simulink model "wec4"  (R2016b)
settings: Solver=ode4  StartTime=0  StopTime=1000  FixedStep=0.005  MaxStep=0.005  RelTol=1e-3  EnableMultiTasking=on
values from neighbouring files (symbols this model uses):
  arAdaptiveLawData = 1/2*zModelSimple.zModelPto.arFreq.*     zModelSimple.zModelPto.arMagnitude./     cos(zModelSimple.zModelPto.arPhase*pi/180+pi/2)    [IMPACT_Control.m]
  arAdaptiveLawDataX = 1/2*zModelSimpleX.zModelPto.arFreq.*         zModelSimpleX.zModelPto.arMagnitude./         cos(zModelSimpleX.zModelPto.arPhase*pi/180+pi/2)    [IMPACT_Control.m]
  arControllerRampGain = [0,0,1,1]    [IMPACT_Control.m]
  arControllerRampTime = [0 rStartRampTime rStartRampTime+rRampTimeLength 8000]    [IMPACT_Control.m]
  arEkfInitialisation = zeros(1,11)    [IMPACT_Control.m]
  arEkfInitialisationX = zeros(1,11)    [IMPACT_Control.m]
  arFrequency = zModelSimple.zModelPto.arFreq    [IMPACT_Control.m]
  arFrequencyRange = zModelSimple.zModelPto.arFreq    [IMPACT_Control.m]
  arFrequencyX = zModelSimpleX.zModelPto.arFreq    [IMPACT_Control.m]
  arImpedance = 1./zModelSimple.zModelPto.arMagnitude./zModelSimple.zModelPto.arFreq    [IMPACT_Control.m]
  arImpedanceX = 1./zModelSimpleX.zModelPto.arMagnitude./zModelSimpleX.zModelPto.arFreq    [IMPACT_Control.m]
  CentralPTOPreload = -1.6113e+07    (= -16113000)    [wecSimInputFile.m]
  F1 = [4.243 2.375 -12.243]    [wecSimInputFile.m]
  F2 = [4.243 -2.375 -12.243]    [wecSimInputFile.m]
  F3 = [-4.243 -2.375 -12.243]    [wecSimInputFile.m]
  F4 = [-4.243 2.375 -12.243]    [wecSimInputFile.m]
  FC = [0 0 -14]    [wecSimInputFile.m]
  iAdaptiveDamping = 0    [wec4IMPACT_Project.m]    (also in IMPACT_Control.m = handles.iAdaptiveDamping; wec1_IMPACT_Project.m; wec2_IMPACT_Project.m; wec3_IMPACT_Project.m)
  iControlType = 2    [wec4IMPACT_Project.m]    (also in IMPACT_Control.m = handles.iControlType; wec1_IMPACT_Project.m = 1; wec2_IMPACT_Project.m = 1; wec3_IMPACT_Project.m = 1)
  iPtoPositionConstraint = 1    [wec4IMPACT_Project.m]    (also in IMPACT_Control.m = handles.iPtoPositionConstraint; wec1_IMPACT_Project.m = 0; wec2_IMPACT_Project.m; wec3_IMPACT_Project.m)
  iSensorNoise = 0    [IMPACT_Control.m]
  m = m+1    (= 2)    [checkParamFile.m]
  PTOrotation = atan((T1(2)-F1(2))/(T1(1)-F1(1)))    [wecSimInputFile.m]
  rCogFloater = -8    [wec4_IMPACT_Model.m]    (also in paramInitial.m = get( handles.edit_rCogFloater, 'String' ); wec1_IMPACT_Model.m = -18; wec2_IMPACT_Model.m = -8.5; wec3_IMPACT_Model.m = -0.7)
  rCogSpar = -36.6    [wec4_IMPACT_Model.m]    (also in paramInitial.m = get( handles.edit_rCogSpar, 'String' ); wec3_IMPACT_Model.m = -21.3; wec3_IMPACT_Model2.m = -21.3)
  rDisplacementLimit = 10.000000    (= 10)    [wec4IMPACT_Project.m]    (also in IMPACT_Control.m = getValue(handles.edit_displacementLimit); wec1_IMPACT_Project.m; wec2_IMPACT_Project.m; wec3_IMPACT_Project.m = 3)
  rDisplacementLimitX = 10.000000    (= 10)    [wec4IMPACT_Project.m]    (also in IMPACT_Control.m = getValue(handles.edit_displacementLimitX); wec1_IMPACT_Project.m = 0; wec2_IMPACT_Project.m; wec3_IMPACT_Project.m = 0)
  rGainForAntiWIndUp = tfControllerDiscrete.rGain    [IMPACT_Control.m]
  rGainForAntiWIndUpX = tfControllerXDiscrete.rGain    [IMPACT_Control.m]
  rMaxForcePto = 300000000.000000    (= 300000000)    [wec4IMPACT_Project.m]    (also in IMPACT_Control.m = getValue(handles.edit_maxForcePto); wec1_IMPACT_Project.m = 1e+15; wec2_IMPACT_Project.m = 1e+15; wec3_IMPACT_Project.m = 1000000000)
  rMinForcePto = -300000000.000000    (= -300000000)    [wec4IMPACT_Project.m]    (also in IMPACT_Control.m = getValue(handles.edit_minForcePto); wec1_IMPACT_Project.m = -1e+15; wec2_IMPACT_Project.m = -1e+15; wec3_IMPACT_Project.m = -1000000000)
  rMooringX = 20000    [wec4_IMPACT_Model.m]    (also in paramInitial.m = get( handles.edit_rMooringX, 'String' ); wec3_IMPACT_Model.m = 10000; wec3_IMPACT_Model2.m = 10000)
  rMooringZ = 10000    [wec4_IMPACT_Model.m]    (also in paramInitial.m = get( handles.edit_rMooringZ, 'String' ); wec3_IMPACT_Model.m = 0; wec3_IMPACT_Model2.m = 0)
  rOutputSampleTime = 0.010000    (= 0.01)    [wec4IMPACT_Project.m]    (also in IMPACT_Control.m = getValue(handles.edit_outputSampleTime); wec1_IMPACT_Project.m; wec2_IMPACT_Project.m; wec3_IMPACT_Project.m)
  rPassiveDampingGain = -604830.000000    (= -604830)    [wec4IMPACT_Project.m]    (also in IMPACT_Control.m = getValue(handles.edit_gainPLD); wec1_IMPACT_Project.m = -214018.1537; wec2_IMPACT_Project.m = -1948070; wec3_IMPACT_Project.m = -519390)
  rPassiveDampingGainX = -278660.000000    (= -278660)    [wec4IMPACT_Project.m]    (also in IMPACT_Control.m = getValue(handles.edit_gainPLDX); wec1_IMPACT_Project.m = 0; wec2_IMPACT_Project.m = 0; wec3_IMPACT_Project.m = 0)
  rTetherPretension = 1.6113e+07    (= 16113000)    [wec4_IMPACT_Model.m]    (also in paramInitial.m = get( handles.edit_rTetherPretension, 'String' ); wec3_IMPACT_Model.m = 0; wec3_IMPACT_Model2.m = 0)
  rTetherSpring = 500000    [wec4_IMPACT_Model.m]    (also in paramInitial.m = get( handles.edit_rTetherSpring, 'String' ); wec3_IMPACT_Model.m = 0; wec3_IMPACT_Model2.m = 0)
  rUpperFrequencyLimit = EKFFloater.upperFreq    [IMPACT_Control.m]
  rXf = 4.243    [wec4AdditionalParams.m]
  rXs = 16.075    [wec4AdditionalParams.m]
  rYf = 2.375    [wec4AdditionalParams.m]
  rYs = 16.075    [wec4AdditionalParams.m]
  rZf = 4.243    [wec4AdditionalParams.m]
  rZs = 2.4350    (= 2.435)    [wec4AdditionalParams.m]
  rZTetherF = 6    [wec4AdditionalParams.m]
  rZTetherS = 2.4350    (= 2.435)    [wec4AdditionalParams.m]
  s = tf('s')    [wec4_IMPACT_Model.m]    (also in IMPACT_Control.m; wec1_IMPACT_Model.m; wec2_IMPACT_Model.m; wec3_IMPACT_Model.m)
  SidePTO1Preload = PreloadPTOCorner    (= 0)    [wecSimInputFile.m]
  SidePTO2Preload = PreloadPTOCorner    (= 0)    [wecSimInputFile.m]
  SidePTO3Preload = PreloadPTOCorner    (= 0)    [wecSimInputFile.m]
  SidePTO4Preload = PreloadPTOCorner    (= 0)    [wecSimInputFile.m]
  simu = simulationClass()    [wecSimInputFile.m]
  T1 = [16.075 16.075 -34.165]    [wecSimInputFile.m]
  T2 = [16.075 -16.075 -34.165]    [wecSimInputFile.m]
  T3 = [-16.075 -16.075 -34.165]    [wecSimInputFile.m]
  T4 = [-16.075 16.075 -34.165]    [wecSimInputFile.m]
  TC = [0 0 -34.165]    [wecSimInputFile.m]
  waves = waveClass('irregular')    [wecSimInputFile.m]
  Z = magPhaseToComplex(zModelTf)    [IMPACT_Control.m]
undefined symbols (not defined in the file or in its folder): arControllerDiscreteDen, arControllerDiscreteNum, arControllerDiscreteXDen, arControllerDiscreteXNum, arExcForceFloaterDen, arExcForceFloaterNum, arExcForceFloaterXDen, arExcForceFloaterXNum, arExcForceSparDen, arExcForceSparNum, arExcForceSparXDen, arExcForceSparXNum, arFexcFloaterDen, arFexcFloaterNum, arFexcFloaterXDen, arFexcFloaterXNum, arFexcSparDen, arFexcSparNum, arFexcSparXDen, arFexcSparXNum, Body, body, constraint, CTTime, deg, Elements, geometry, IRKB, kg, lenJ, mooring, N, pto, rAccelerationGainFloater, rAccelerationGainFloaterX, rAccelerationGainSpar, rAccelerationGainSparX, rad, rBuoyancyGainFloater, rBuoyancyGainFloaterX, rBuoyancyGainSpar, rBuoyancyGainSparX, rDampingGainFloater, rDampingGainFloaterX, rDampingGainSpar, rDampingGainSparX, Rigid, rMaxFocePto, wec4_float, wec4_reactor, WECSim_Lib, X, Y
libraries: nesl_utility x380, sm_lib x170, vrlib x91, simulink x12, WECSim_Lib x4
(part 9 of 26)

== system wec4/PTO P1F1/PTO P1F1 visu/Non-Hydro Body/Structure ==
  Total Force : Inport
  Body Properties : sm_lib/Body Elements/Solid  InertiaType=Custom  Mass=body.mass  MassUnits=kg  CenterOfMass=[0 0 0]  CenterOfMassUnits=m  MomentsOfInertia=body.momOfInertia  MomentsOfInertiaUnits=kg*m^2  ProductsOfInertia=[0 0 0]  ProductsOfInertiaUnits=kg*m^2  DensityBased=on  Density=1000  DensityUnits=kg/(m^3)  DoExposeReferenceFrame=on  SerializedFrames=<Frames/>  GraphicType=FromGeometry  MarkerShape=Sphere  MarkerSize=10  MarkerSizeUnits=m  GraphicVisPropType=SimpleVisualProperties  GraphicDiffuseColor=body.viz.color  GraphicSpecularColor=[0.5 0.5 0.5 1.0]  GraphicAmbientColor=[0.15 0.15 0.15 1.0]  GraphicEmissiveColor=[0.0 0.0 0.0 1.0]  GraphicShininess=75  GraphicOpacity=body.viz.opacity  GeometryShape=FromFile  RectangleSize=[1 1]  RectangleSizeUnits=m  BrickDimensions=[1 1 1]  BrickDimensionUnits=m  CylinderRadius=1  CylinderRadiusUnits=m  CylinderLength=1  CylinderLengthUnits=m  SphereRadius=1  SphereRadiusUnits=m  EllipsoidRadii=[1 1 1]  EllipsoidRadiiUnits=m  ExtrusionCrossSection=[1 1; -1 1; -1 -1; 1 -1]  ExtrusionCrossSectionUnits=m  ExtrusionLength=1  ExtrusionLengthUnits=m  PolygonNumSides=3  PolygonOuterRadius=1  PolygonOuterRadiusUnits=m  ExtGeomFileType=STL  ExtGeomFileName=.\geometry\pto_visu.stl  ExtGeomFileUnits=m  RevolutionCrossSection=[1 1; 1 -1; 2 -1; 2 1]  RevolutionCrossSectionUnits=m  RevolutionExtent=Full  RevolutionAngle=180  RevolutionAngleUnits=deg
  External Force and Torque : sm_lib/Forces and Torques/External Force and Torque  ForceResolutionFrame=World  EnableForceX=off  EnableForceY=off  EnableForceZ=off  EnableForce=on  TorqueResolutionFrame=World  EnableTorqueX=off  EnableTorqueY=off  EnableTorqueZ=off  EnableTorque=on
  Motion Sensor : Subsystem
  Rigid Transform (Setup CG) : sm_lib/Frames and Transforms/Rigid Transform  TranslationMethod=Cartesian  TranslationStandardOffset=0  TranslationLengthUnit=m  TranslationStandardAxis=+Z  TranslationCartesianOffset=body.cg  TranslationROffset=0  TranslationROffsetUnits=m  TranslationZOffset=0  TranslationZOffsetUnits=m  TranslationThetaOffset=0  TranslationThetaOffsetUnits=deg  RotationMethod=None  RotationAngleUnits=rad  RotationStandardAxis=+Y  RotationAngle=0.05  RotationArbitraryAxis=[0.57735026918962584 0.57735026918962584 0.57735026918962584]  FollAlignAxisA=+X  BaseAlignAxisA=+Y  FollAlignAxisB=+Y  BaseAlignAxisB=+Z  RotationSequenceAxes=FollowerAxes  RotationSequence=XYX  RotationSequenceAngles=[0 0 0]  RotationSequenceAnglesUnits=deg  RotationMatrix=[1 0 0; 0 1 0; 0 0 1]
  Rigid Transform (Setup Initial Disp) : sm_lib/Frames and Transforms/Rigid Transform  TranslationMethod=Cartesian  TranslationStandardOffset=0  TranslationLengthUnit=m  TranslationStandardAxis=+Z  TranslationCartesianOffset=body.initDisp.initLinDisp  TranslationROffset=0  TranslationROffsetUnits=m  TranslationZOffset=0  TranslationZOffsetUnits=m  TranslationThetaOffset=0  TranslationThetaOffsetUnits=deg  RotationMethod=ArbitraryAxis  RotationAngleUnits=rad  RotationStandardAxis=+Y  RotationAngle=body.initDisp.initAngularDispAngle  RotationArbitraryAxis=body.initDisp.initAngularDispAxis  FollAlignAxisA=+X  BaseAlignAxisA=+Y  FollAlignAxisB=+Y  BaseAlignAxisB=+Z  RotationSequenceAxes=FollowerAxes  RotationSequence=XYX  RotationSequenceAngles=[0 0 0]  RotationSequenceAnglesUnits=deg  RotationMatrix=[1 0 0; 0 1 0; 0 0 1]
  Selector : Selector  InputPortWidth=6  IndexOptions=Index vector (dialog)  Indices=[1:3]  OutputSizes=1
  Selector1 : Selector  InputPortWidth=6  IndexOptions=Index vector (dialog)  Indices=[4:6]  OutputSizes=1
  Simulink-PS Converter1 : nesl_utility/Simulink-PS Converter  PhysicalDomain=network_engine_domain  SubClassName=ps_input  LeftPortType=input  RightPortType=output  PseudoPeriodic=off  Frequencies=[]  NoiseDistribution=none  NoiseParameters=[]  Unit=1  AffineConversion=off  InputFiltering=off  SimscapeFilterOrder=1  InputFilterTimeConstant=0.001  UdotUserProvided=1
  Simulink-PS Converter2 : nesl_utility/Simulink-PS Converter  PhysicalDomain=network_engine_domain  SubClassName=ps_input  LeftPortType=input  RightPortType=output  PseudoPeriodic=off  Frequencies=[]  NoiseDistribution=none  NoiseParameters=[]  Unit=1  AffineConversion=off  InputFiltering=off  SimscapeFilterOrder=1  InputFilterTimeConstant=0.001  UdotUserProvided=1
  World Frame : sm_lib/Frames and Transforms/World Frame
  Conn Free Surface : PMIOPort  Port=1  Side=Right
  Response : Outport
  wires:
  Total Force/1 -> Selector1/1, Selector/1
  Selector/1 -> Simulink-PS Converter1/1
  Selector1/1 -> Simulink-PS Converter2/1
  Motion Sensor/1(Response) -> Response/1
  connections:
  External Force and Torque/LConn1 -- Simulink-PS Converter1/RConn1
  External Force and Torque/LConn2 -- Simulink-PS Converter2/RConn1
  Rigid Transform (Setup Initial Disp)/RConn1 -- Body Properties/RConn1 -- External Force and Torque/RConn1 -- Motion Sensor/RConn1
  Conn Free Surface/RConn1 -- Rigid Transform (Setup CG)/LConn1
  Rigid Transform (Setup Initial Disp)/LConn1 -- Rigid Transform (Setup CG)/RConn1
  World Frame/RConn1 -- Motion Sensor/LConn1

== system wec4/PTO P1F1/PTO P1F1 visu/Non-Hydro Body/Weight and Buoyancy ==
  Add1 : Sum  Inputs=+-
  Assignment (Add Net Bouyancy Force to Z-Direction) : Assignment  IndexOptions=Index vector (dialog)  Indices=3  OutputSizes=1
  Body Mass : Constant  Value=body.mass
  Constant1 : Constant  Value=[0 0 0 0 0 0]
  Gravity : Constant  Value=simu.g
  Product : Product
  Product1 : Product  Inputs=3
  Volume : Constant  Value=body.dispVol
  Water Density : Constant  Value=simu.rho
  Out1 : Outport
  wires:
  Add1/1 -> Assignment (Add Net Bouyancy Force to Z-Direction)/2
  Product1/1 -> Add1/2  "F_Buoyancy"
  Product/1 -> Add1/1  "F_Gravity"
  Water Density/1 -> Product1/1  "rho"
  Gravity/1 -> Product/1, Product1/2  "g"
  Volume/1 -> Product1/3  "Vol"
  Assignment (Add Net Bouyancy Force to Z-Direction)/1 -> Out1/1  "F_Restoring"
  Constant1/1 -> Assignment (Add Net Bouyancy Force to Z-Direction)/1
  Body Mass/1 -> Product/2  "m"

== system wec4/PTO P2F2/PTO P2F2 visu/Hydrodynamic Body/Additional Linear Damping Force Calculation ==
  Velocity : Inport
  Additional Linear Damping Matrix (diagonal) : Constant  Value=body.hydroForce.linearDamping
  Product1 : Product  Multiplication=Matrix(*)
  F_LinearDamping : Outport
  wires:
  Velocity/1 -> Product1/2  "v"
  Product1/1 -> F_LinearDamping/1  "F_LinearDamping"
  Additional Linear Damping Matrix (diagonal)/1 -> Product1/1  "C"

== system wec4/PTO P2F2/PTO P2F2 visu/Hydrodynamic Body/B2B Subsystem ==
  note: 1) Add Subsystem or Model blocks as valid variant choices. 2) You cannot connect blocks at this level. At simulation, connectivity is automatically determined, based on the active variant and port name matching.
  vel_in : Inport
  acc_in : Inport  Port=2
  B2B : Subsystem  VariantControl=sv_B2B
  noB2B : Subsystem  VariantControl=sv_noB2B
  vel : Outport
  acc : Outport  Port=2

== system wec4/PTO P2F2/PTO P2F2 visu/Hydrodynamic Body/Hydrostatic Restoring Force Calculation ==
  Displacement : Inport
  Wave Elv : Inport  Port=2
  Add : Sum  Inputs=+-
  Center of Gravity : Constant  Value=body.cg
  Constant : Constant  Value=[0 0 0]
  Linear and Nonlinear Restoring Force Variant Subsystem : Subsystem  Variant=on
  Mux : Mux  Inputs=2
  F_Restoring : Outport
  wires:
  Add/1 -> Linear and Nonlinear Restoring Force Variant Subsystem/1(In1)  "x_cg"
  Wave Elv/1 -> Linear and Nonlinear Restoring Force Variant Subsystem/2(In2)
  Constant/1 -> Mux/2
  Center of Gravity/1 -> Mux/1  "cg"
  Mux/1 -> Add/2
  Linear and Nonlinear Restoring Force Variant Subsystem/1(Out1) -> F_Restoring/1  "F_Restoring"
  Displacement/1 -> Add/1  "x"

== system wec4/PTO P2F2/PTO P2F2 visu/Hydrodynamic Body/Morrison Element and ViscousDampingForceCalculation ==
  Displacement : Inport
  Acceleration : Inport  Port=2
  Velocity : Inport  Port=3
  Time : Inport  Port=4
  Abs1 : Abs
  Morrison Element Variant Subsystem : Subsystem  Variant=on
  Product : Product
  Product1 : Product  Multiplication=Matrix(*)
  Transport Delay : TransportDelay  DelayTime=10e-8
  "VisSum " : Sum  Inputs=+-
  "Viscous Damping Matrix (diagonal) " : Constant  Value=body.hydroForce.visDrag
  F_MorrisonAndViscous : Outport
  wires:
  Time/1 -> Morrison Element Variant Subsystem/4(time)
  Morrison Element Variant Subsystem/1(morison_force) -> "VisSum "/2
  Displacement/1 -> Morrison Element Variant Subsystem/1(displacement)
  Product/1 -> Product1/2  "v * |v|"
  "Viscous Damping Matrix (diagonal) "/1 -> Product1/1  "0.5 * cd * rho *A"
  Product1/1 -> "VisSum "/1
  Abs1/1 -> Product/2
  Acceleration/1 -> Transport Delay/1
  Transport Delay/1 -> Morrison Element Variant Subsystem/3(acceleration)
  "VisSum "/1 -> F_MorrisonAndViscous/1  "F_MorrisonAndViscous"
  Velocity/1 -> Abs1/1, Product/1, Morrison Element Variant Subsystem/2(velocity)

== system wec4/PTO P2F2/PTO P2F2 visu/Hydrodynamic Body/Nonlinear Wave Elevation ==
  Displacement : Inport
  Time : Inport  Port=2
  Add : Sum  Inputs=+-
  Center of Gravity : Constant  Value=body.cg
  Constant : Constant  Value=[0 0 0]
  Linear or Instantaneous Free Surface : Subsystem  Variant=on
  Mux : Mux  Inputs=2
  Wave Elevation : Outport
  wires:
  Time/1 -> Linear or Instantaneous Free Surface/2(In2)
  Constant/1 -> Mux/2
  Center of Gravity/1 -> Mux/1  "cg"
  Mux/1 -> Add/2
  Add/1 -> Linear or Instantaneous Free Surface/1(In1)  "x_cg"
  Linear or Instantaneous Free Surface/1(Out1) -> Wave Elevation/1
  Displacement/1 -> Add/1  "x"

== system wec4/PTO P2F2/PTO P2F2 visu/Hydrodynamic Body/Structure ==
  Total Force : Inport
  Body Properties : sm_lib/Body Elements/Solid  InertiaType=Custom  Mass=body.mass  MassUnits=kg  CenterOfMass=[0 0 0]  CenterOfMassUnits=m  MomentsOfInertia=body.momOfInertia  MomentsOfInertiaUnits=kg*m^2  ProductsOfInertia=[0 0 0]  ProductsOfInertiaUnits=kg*m^2  DensityBased=on  Density=1000  DensityUnits=kg/(m^3)  DoExposeReferenceFrame=on  SerializedFrames=<Frames/>  GraphicType=FromGeometry  MarkerShape=Sphere  MarkerSize=10  MarkerSizeUnits=m  GraphicVisPropType=SimpleVisualProperties  GraphicDiffuseColor=body.viz.color  GraphicSpecularColor=[0.5 0.5 0.5 1.0]  GraphicAmbientColor=[0.15 0.15 0.15 1.0]  GraphicEmissiveColor=[0.0 0.0 0.0 1.0]  GraphicShininess=75  GraphicOpacity=body.viz.opacity  GeometryShape=FromFile  RectangleSize=[1 1]  RectangleSizeUnits=m  BrickDimensions=[1 1 1]  BrickDimensionUnits=m  CylinderRadius=1  CylinderRadiusUnits=m  CylinderLength=1  CylinderLengthUnits=m  SphereRadius=1  SphereRadiusUnits=m  EllipsoidRadii=[1 1 1]  EllipsoidRadiiUnits=m  ExtrusionCrossSection=[1 1; -1 1; -1 -1; 1 -1]  ExtrusionCrossSectionUnits=m  ExtrusionLength=1  ExtrusionLengthUnits=m  PolygonNumSides=3  PolygonOuterRadius=1  PolygonOuterRadiusUnits=m  ExtGeomFileType=STL  ExtGeomFileName=.\geometry\pto_visu.stl  ExtGeomFileUnits=m  RevolutionCrossSection=[1 1; 1 -1; 2 -1; 2 1]  RevolutionCrossSectionUnits=m  RevolutionExtent=Full  RevolutionAngle=180  RevolutionAngleUnits=deg
  External Force and Torque : sm_lib/Forces and Torques/External Force and Torque  ForceResolutionFrame=World  EnableForceX=off  EnableForceY=off  EnableForceZ=off  EnableForce=on  TorqueResolutionFrame=World  EnableTorqueX=off  EnableTorqueY=off  EnableTorqueZ=off  EnableTorque=on
  Motion Sensor : Subsystem
  Rigid Transform (Setup CG) : sm_lib/Frames and Transforms/Rigid Transform  TranslationMethod=Cartesian  TranslationStandardOffset=0  TranslationLengthUnit=m  TranslationStandardAxis=+Z  TranslationCartesianOffset=body.cg  TranslationROffset=0  TranslationROffsetUnits=m  TranslationZOffset=0  TranslationZOffsetUnits=m  TranslationThetaOffset=0  TranslationThetaOffsetUnits=deg  RotationMethod=None  RotationAngleUnits=rad  RotationStandardAxis=+Y  RotationAngle=0.05  RotationArbitraryAxis=[0.57735026918962584 0.57735026918962584 0.57735026918962584]  FollAlignAxisA=+X  BaseAlignAxisA=+Y  FollAlignAxisB=+Y  BaseAlignAxisB=+Z  RotationSequenceAxes=FollowerAxes  RotationSequence=XYX  RotationSequenceAngles=[0 0 0]  RotationSequenceAnglesUnits=deg  RotationMatrix=[1 0 0; 0 1 0; 0 0 1]
  Rigid Transform (Setup Initial Disp) : sm_lib/Frames and Transforms/Rigid Transform  TranslationMethod=Cartesian  TranslationStandardOffset=0  TranslationLengthUnit=m  TranslationStandardAxis=+Z  TranslationCartesianOffset=body.initDisp.initLinDisp  TranslationROffset=0  TranslationROffsetUnits=m  TranslationZOffset=0  TranslationZOffsetUnits=m  TranslationThetaOffset=0  TranslationThetaOffsetUnits=deg  RotationMethod=ArbitraryAxis  RotationAngleUnits=rad  RotationStandardAxis=+Y  RotationAngle=body.initDisp.initAngularDispAngle  RotationArbitraryAxis=body.initDisp.initAngularDispAxis  FollAlignAxisA=+X  BaseAlignAxisA=+Y  FollAlignAxisB=+Y  BaseAlignAxisB=+Z  RotationSequenceAxes=FollowerAxes  RotationSequence=XYX  RotationSequenceAngles=[0 0 0]  RotationSequenceAnglesUnits=deg  RotationMatrix=[1 0 0; 0 1 0; 0 0 1]
  Selector : Selector  InputPortWidth=6  IndexOptions=Index vector (dialog)  Indices=[1:3]  OutputSizes=1
  Selector1 : Selector  InputPortWidth=6  IndexOptions=Index vector (dialog)  Indices=[4:6]  OutputSizes=1
  Simulink-PS Converter1 : nesl_utility/Simulink-PS Converter  PhysicalDomain=network_engine_domain  SubClassName=ps_input  LeftPortType=input  RightPortType=output  PseudoPeriodic=off  Frequencies=[]  NoiseDistribution=none  NoiseParameters=[]  Unit=1  AffineConversion=off  InputFiltering=off  SimscapeFilterOrder=1  InputFilterTimeConstant=0.001  UdotUserProvided=1
  Simulink-PS Converter2 : nesl_utility/Simulink-PS Converter  PhysicalDomain=network_engine_domain  SubClassName=ps_input  LeftPortType=input  RightPortType=output  PseudoPeriodic=off  Frequencies=[]  NoiseDistribution=none  NoiseParameters=[]  Unit=1  AffineConversion=off  InputFiltering=off  SimscapeFilterOrder=1  InputFilterTimeConstant=0.001  UdotUserProvided=1
  World Frame : sm_lib/Frames and Transforms/World Frame
  Conn Free Surface : PMIOPort  Port=1  Side=Right
  Response : Outport
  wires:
  Total Force/1 -> Selector1/1, Selector/1
  Selector/1 -> Simulink-PS Converter1/1
  Selector1/1 -> Simulink-PS Converter2/1
  Motion Sensor/1(Response) -> Response/1
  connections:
  External Force and Torque/LConn1 -- Simulink-PS Converter1/RConn1
  External Force and Torque/LConn2 -- Simulink-PS Converter2/RConn1
  Rigid Transform (Setup Initial Disp)/RConn1 -- Body Properties/RConn1 -- External Force and Torque/RConn1 -- Motion Sensor/RConn1
  Conn Free Surface/RConn1 -- Rigid Transform (Setup CG)/LConn1
  Rigid Transform (Setup Initial Disp)/LConn1 -- Rigid Transform (Setup CG)/RConn1
  World Frame/RConn1 -- Motion Sensor/LConn1

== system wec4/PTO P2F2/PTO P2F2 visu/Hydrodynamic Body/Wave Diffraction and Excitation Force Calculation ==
  Time : Inport
  Displacement : Inport  Port=2
  WaveElv : Inport  Port=3
  Add : Sum
  If2 : If  NumInputs=2  IfExpression=u1 < u2
  Linear Wave Excitation Force Variant Subsystem : Subsystem  Variant=on
  Merge1 : Merge
  No Ramp Function : Subsystem  TreatAsAtomicUnit=on
  Nonlinear FK Force Variant Subsystem : Subsystem  Variant=on
  Product : Product
  Ramp Function : Subsystem  TreatAsAtomicUnit=on
  Ramp Function Time : Constant  Value=simu.rampTime
  F_Excitation : Outport  PortDimensions=6
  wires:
  Nonlinear FK Force Variant Subsystem/1(Out1) -> Add/2
  Linear Wave Excitation Force Variant Subsystem/1(Out1) -> Add/1
  WaveElv/1 -> Nonlinear FK Force Variant Subsystem/3(In3)
  Displacement/1 -> Nonlinear FK Force Variant Subsystem/2(In2)
  Product/1 -> F_Excitation/1  "F_Excitation"
  Add/1 -> Product/2  "F_wave"
  Time/1 -> If2/1, Ramp Function/1(Time), Nonlinear FK Force Variant Subsystem/1(In1), Linear Wave Excitation Force Variant Subsystem/1(In1)
  Merge1/1 -> Product/1  "R"
  Ramp Function Time/1 -> If2/2
  If2/2 -> No Ramp Function/Action
  If2/1 -> Ramp Function/Action
  Ramp Function/1(R) -> Merge1/1
  No Ramp Function/1(R) -> Merge1/2

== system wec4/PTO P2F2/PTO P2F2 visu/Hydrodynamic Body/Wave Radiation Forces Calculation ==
  Velocity : Inport
  Acceleration : Inport  Port=2
  Time : Inport  Port=3
  Added Mass Matrix : Constant  Value=body.hydroForce.fAddedMass
  Product1 : Product  Multiplication=Matrix(*)
  SS CI and Constant-Damping-CoeVariant Subsystem : Subsystem  Variant=on
  Transport Delay : TransportDelay  DelayTime=10e-8
  F_RadiationDamping : Outport
  F_AddedMass : Outport  Port=2
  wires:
  Time/1 -> SS CI and Constant-Damping-CoeVariant Subsystem/2(In2)
  Acceleration/1 -> Transport Delay/1
  Transport Delay/1 -> Product1/2
  SS CI and Constant-Damping-CoeVariant Subsystem/1(Out1) -> F_RadiationDamping/1  "F_RadiationDamping"
  Velocity/1 -> SS CI and Constant-Damping-CoeVariant Subsystem/1(In1)
  Product1/1 -> F_AddedMass/1  "F_AddedMass"
  Added Mass Matrix/1 -> Product1/1

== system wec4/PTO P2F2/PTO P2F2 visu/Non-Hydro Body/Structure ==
  Total Force : Inport
  Body Properties : sm_lib/Body Elements/Solid  InertiaType=Custom  Mass=body.mass  MassUnits=kg  CenterOfMass=[0 0 0]  CenterOfMassUnits=m  MomentsOfInertia=body.momOfInertia  MomentsOfInertiaUnits=kg*m^2  ProductsOfInertia=[0 0 0]  ProductsOfInertiaUnits=kg*m^2  DensityBased=on  Density=1000  DensityUnits=kg/(m^3)  DoExposeReferenceFrame=on  SerializedFrames=<Frames/>  GraphicType=FromGeometry  MarkerShape=Sphere  MarkerSize=10  MarkerSizeUnits=m  GraphicVisPropType=SimpleVisualProperties  GraphicDiffuseColor=body.viz.color  GraphicSpecularColor=[0.5 0.5 0.5 1.0]  GraphicAmbientColor=[0.15 0.15 0.15 1.0]  GraphicEmissiveColor=[0.0 0.0 0.0 1.0]  GraphicShininess=75  GraphicOpacity=body.viz.opacity  GeometryShape=FromFile  RectangleSize=[1 1]  RectangleSizeUnits=m  BrickDimensions=[1 1 1]  BrickDimensionUnits=m  CylinderRadius=1  CylinderRadiusUnits=m  CylinderLength=1  CylinderLengthUnits=m  SphereRadius=1  SphereRadiusUnits=m  EllipsoidRadii=[1 1 1]  EllipsoidRadiiUnits=m  ExtrusionCrossSection=[1 1; -1 1; -1 -1; 1 -1]  ExtrusionCrossSectionUnits=m  ExtrusionLength=1  ExtrusionLengthUnits=m  PolygonNumSides=3  PolygonOuterRadius=1  PolygonOuterRadiusUnits=m  ExtGeomFileType=STL  ExtGeomFileName=.\geometry\pto_visu.stl  ExtGeomFileUnits=m  RevolutionCrossSection=[1 1; 1 -1; 2 -1; 2 1]  RevolutionCrossSectionUnits=m  RevolutionExtent=Full  RevolutionAngle=180  RevolutionAngleUnits=deg
  External Force and Torque : sm_lib/Forces and Torques/External Force and Torque  ForceResolutionFrame=World  EnableForceX=off  EnableForceY=off  EnableForceZ=off  EnableForce=on  TorqueResolutionFrame=World  EnableTorqueX=off  EnableTorqueY=off  EnableTorqueZ=off  EnableTorque=on
  Motion Sensor : Subsystem
  Rigid Transform (Setup CG) : sm_lib/Frames and Transforms/Rigid Transform  TranslationMethod=Cartesian  TranslationStandardOffset=0  TranslationLengthUnit=m  TranslationStandardAxis=+Z  TranslationCartesianOffset=body.cg  TranslationROffset=0  TranslationROffsetUnits=m  TranslationZOffset=0  TranslationZOffsetUnits=m  TranslationThetaOffset=0  TranslationThetaOffsetUnits=deg  RotationMethod=None  RotationAngleUnits=rad  RotationStandardAxis=+Y  RotationAngle=0.05  RotationArbitraryAxis=[0.57735026918962584 0.57735026918962584 0.57735026918962584]  FollAlignAxisA=+X  BaseAlignAxisA=+Y  FollAlignAxisB=+Y  BaseAlignAxisB=+Z  RotationSequenceAxes=FollowerAxes  RotationSequence=XYX  RotationSequenceAngles=[0 0 0]  RotationSequenceAnglesUnits=deg  RotationMatrix=[1 0 0; 0 1 0; 0 0 1]
  Rigid Transform (Setup Initial Disp) : sm_lib/Frames and Transforms/Rigid Transform  TranslationMethod=Cartesian  TranslationStandardOffset=0  TranslationLengthUnit=m  TranslationStandardAxis=+Z  TranslationCartesianOffset=body.initDisp.initLinDisp  TranslationROffset=0  TranslationROffsetUnits=m  TranslationZOffset=0  TranslationZOffsetUnits=m  TranslationThetaOffset=0  TranslationThetaOffsetUnits=deg  RotationMethod=ArbitraryAxis  RotationAngleUnits=rad  RotationStandardAxis=+Y  RotationAngle=body.initDisp.initAngularDispAngle  RotationArbitraryAxis=body.initDisp.initAngularDispAxis  FollAlignAxisA=+X  BaseAlignAxisA=+Y  FollAlignAxisB=+Y  BaseAlignAxisB=+Z  RotationSequenceAxes=FollowerAxes  RotationSequence=XYX  RotationSequenceAngles=[0 0 0]  RotationSequenceAnglesUnits=deg  RotationMatrix=[1 0 0; 0 1 0; 0 0 1]
  Selector : Selector  InputPortWidth=6  IndexOptions=Index vector (dialog)  Indices=[1:3]  OutputSizes=1
  Selector1 : Selector  InputPortWidth=6  IndexOptions=Index vector (dialog)  Indices=[4:6]  OutputSizes=1
  Simulink-PS Converter1 : nesl_utility/Simulink-PS Converter  PhysicalDomain=network_engine_domain  SubClassName=ps_input  LeftPortType=input  RightPortType=output  PseudoPeriodic=off  Frequencies=[]  NoiseDistribution=none  NoiseParameters=[]  Unit=1  AffineConversion=off  InputFiltering=off  SimscapeFilterOrder=1  InputFilterTimeConstant=0.001  UdotUserProvided=1
  Simulink-PS Converter2 : nesl_utility/Simulink-PS Converter  PhysicalDomain=network_engine_domain  SubClassName=ps_input  LeftPortType=input  RightPortType=output  PseudoPeriodic=off  Frequencies=[]  NoiseDistribution=none  NoiseParameters=[]  Unit=1  AffineConversion=off  InputFiltering=off  SimscapeFilterOrder=1  InputFilterTimeConstant=0.001  UdotUserProvided=1
  World Frame : sm_lib/Frames and Transforms/World Frame
  Conn Free Surface : PMIOPort  Port=1  Side=Right
  Response : Outport
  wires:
  Total Force/1 -> Selector1/1, Selector/1
  Selector/1 -> Simulink-PS Converter1/1
  Selector1/1 -> Simulink-PS Converter2/1
  Motion Sensor/1(Response) -> Response/1
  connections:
  External Force and Torque/LConn1 -- Simulink-PS Converter1/RConn1
  External Force and Torque/LConn2 -- Simulink-PS Converter2/RConn1
  Rigid Transform (Setup Initial Disp)/RConn1 -- Body Properties/RConn1 -- External Force and Torque/RConn1 -- Motion Sensor/RConn1
  Conn Free Surface/RConn1 -- Rigid Transform (Setup CG)/LConn1
  Rigid Transform (Setup Initial Disp)/LConn1 -- Rigid Transform (Setup CG)/RConn1
  World Frame/RConn1 -- Motion Sensor/LConn1

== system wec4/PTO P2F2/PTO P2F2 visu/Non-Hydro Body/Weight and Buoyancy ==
  Add1 : Sum  Inputs=+-
  Assignment (Add Net Bouyancy Force to Z-Direction) : Assignment  IndexOptions=Index vector (dialog)  Indices=3  OutputSizes=1
  Body Mass : Constant  Value=body.mass
  Constant1 : Constant  Value=[0 0 0 0 0 0]
  Gravity : Constant  Value=simu.g
  Product : Product
  Product1 : Product  Inputs=3
  Volume : Constant  Value=body.dispVol
  Water Density : Constant  Value=simu.rho
  Out1 : Outport
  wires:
  Add1/1 -> Assignment (Add Net Bouyancy Force to Z-Direction)/2
  Product1/1 -> Add1/2  "F_Buoyancy"
  Product/1 -> Add1/1  "F_Gravity"
  Water Density/1 -> Product1/1  "rho"
  Gravity/1 -> Product/1, Product1/2  "g"
  Volume/1 -> Product1/3  "Vol"
  Assignment (Add Net Bouyancy Force to Z-Direction)/1 -> Out1/1  "F_Restoring"
  Constant1/1 -> Assignment (Add Net Bouyancy Force to Z-Direction)/1
  Body Mass/1 -> Product/2  "m"

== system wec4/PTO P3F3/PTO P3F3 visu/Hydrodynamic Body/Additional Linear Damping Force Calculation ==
  Velocity : Inport
  Additional Linear Damping Matrix (diagonal) : Constant  Value=body.hydroForce.linearDamping
  Product1 : Product  Multiplication=Matrix(*)
  F_LinearDamping : Outport
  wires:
  Velocity/1 -> Product1/2  "v"
  Product1/1 -> F_LinearDamping/1  "F_LinearDamping"
  Additional Linear Damping Matrix (diagonal)/1 -> Product1/1  "C"

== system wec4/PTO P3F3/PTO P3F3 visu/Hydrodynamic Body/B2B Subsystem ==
  note: 1) Add Subsystem or Model blocks as valid variant choices. 2) You cannot connect blocks at this level. At simulation, connectivity is automatically determined, based on the active variant and port name matching.
  vel_in : Inport
  acc_in : Inport  Port=2
  B2B : Subsystem  VariantControl=sv_B2B
  noB2B : Subsystem  VariantControl=sv_noB2B
  vel : Outport
  acc : Outport  Port=2

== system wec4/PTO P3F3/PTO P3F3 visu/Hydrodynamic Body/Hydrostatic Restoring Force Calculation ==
  Displacement : Inport
  Wave Elv : Inport  Port=2
  Add : Sum  Inputs=+-
  Center of Gravity : Constant  Value=body.cg
  Constant : Constant  Value=[0 0 0]
  Linear and Nonlinear Restoring Force Variant Subsystem : Subsystem  Variant=on
  Mux : Mux  Inputs=2
  F_Restoring : Outport
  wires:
  Add/1 -> Linear and Nonlinear Restoring Force Variant Subsystem/1(In1)  "x_cg"
  Wave Elv/1 -> Linear and Nonlinear Restoring Force Variant Subsystem/2(In2)
  Constant/1 -> Mux/2
  Center of Gravity/1 -> Mux/1  "cg"
  Mux/1 -> Add/2
  Linear and Nonlinear Restoring Force Variant Subsystem/1(Out1) -> F_Restoring/1  "F_Restoring"
  Displacement/1 -> Add/1  "x"

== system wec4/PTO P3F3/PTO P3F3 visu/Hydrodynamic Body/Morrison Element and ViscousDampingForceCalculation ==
  Displacement : Inport
  Acceleration : Inport  Port=2
  Velocity : Inport  Port=3
  Time : Inport  Port=4
  Abs1 : Abs
  Morrison Element Variant Subsystem : Subsystem  Variant=on
  Product : Product
  Product1 : Product  Multiplication=Matrix(*)
  Transport Delay : TransportDelay  DelayTime=10e-8
  "VisSum " : Sum  Inputs=+-
  "Viscous Damping Matrix (diagonal) " : Constant  Value=body.hydroForce.visDrag
  F_MorrisonAndViscous : Outport
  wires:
  Time/1 -> Morrison Element Variant Subsystem/4(time)
  Morrison Element Variant Subsystem/1(morison_force) -> "VisSum "/2
  Displacement/1 -> Morrison Element Variant Subsystem/1(displacement)
  Product/1 -> Product1/2  "v * |v|"
  "Viscous Damping Matrix (diagonal) "/1 -> Product1/1  "0.5 * cd * rho *A"
  Product1/1 -> "VisSum "/1
  Abs1/1 -> Product/2
  Acceleration/1 -> Transport Delay/1
  Transport Delay/1 -> Morrison Element Variant Subsystem/3(acceleration)
  "VisSum "/1 -> F_MorrisonAndViscous/1  "F_MorrisonAndViscous"
  Velocity/1 -> Abs1/1, Product/1, Morrison Element Variant Subsystem/2(velocity)

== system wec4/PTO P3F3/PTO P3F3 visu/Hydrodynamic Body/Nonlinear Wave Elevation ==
  Displacement : Inport
  Time : Inport  Port=2
  Add : Sum  Inputs=+-
  Center of Gravity : Constant  Value=body.cg
  Constant : Constant  Value=[0 0 0]
  Linear or Instantaneous Free Surface : Subsystem  Variant=on
  Mux : Mux  Inputs=2
  Wave Elevation : Outport
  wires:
  Time/1 -> Linear or Instantaneous Free Surface/2(In2)
  Constant/1 -> Mux/2
  Center of Gravity/1 -> Mux/1  "cg"
  Mux/1 -> Add/2
  Add/1 -> Linear or Instantaneous Free Surface/1(In1)  "x_cg"
  Linear or Instantaneous Free Surface/1(Out1) -> Wave Elevation/1
  Displacement/1 -> Add/1  "x"

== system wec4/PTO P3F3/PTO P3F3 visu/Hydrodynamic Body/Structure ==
  Total Force : Inport
  Body Properties : sm_lib/Body Elements/Solid  InertiaType=Custom  Mass=body.mass  MassUnits=kg  CenterOfMass=[0 0 0]  CenterOfMassUnits=m  MomentsOfInertia=body.momOfInertia  MomentsOfInertiaUnits=kg*m^2  ProductsOfInertia=[0 0 0]  ProductsOfInertiaUnits=kg*m^2  DensityBased=on  Density=1000  DensityUnits=kg/(m^3)  DoExposeReferenceFrame=on  SerializedFrames=<Frames/>  GraphicType=FromGeometry  MarkerShape=Sphere  MarkerSize=10  MarkerSizeUnits=m  GraphicVisPropType=SimpleVisualProperties  GraphicDiffuseColor=body.viz.color  GraphicSpecularColor=[0.5 0.5 0.5 1.0]  GraphicAmbientColor=[0.15 0.15 0.15 1.0]  GraphicEmissiveColor=[0.0 0.0 0.0 1.0]  GraphicShininess=75  GraphicOpacity=body.viz.opacity  GeometryShape=FromFile  RectangleSize=[1 1]  RectangleSizeUnits=m  BrickDimensions=[1 1 1]  BrickDimensionUnits=m  CylinderRadius=1  CylinderRadiusUnits=m  CylinderLength=1  CylinderLengthUnits=m  SphereRadius=1  SphereRadiusUnits=m  EllipsoidRadii=[1 1 1]  EllipsoidRadiiUnits=m  ExtrusionCrossSection=[1 1; -1 1; -1 -1; 1 -1]  ExtrusionCrossSectionUnits=m  ExtrusionLength=1  ExtrusionLengthUnits=m  PolygonNumSides=3  PolygonOuterRadius=1  PolygonOuterRadiusUnits=m  ExtGeomFileType=STL  ExtGeomFileName=.\geometry\pto_visu.stl  ExtGeomFileUnits=m  RevolutionCrossSection=[1 1; 1 -1; 2 -1; 2 1]  RevolutionCrossSectionUnits=m  RevolutionExtent=Full  RevolutionAngle=180  RevolutionAngleUnits=deg
  External Force and Torque : sm_lib/Forces and Torques/External Force and Torque  ForceResolutionFrame=World  EnableForceX=off  EnableForceY=off  EnableForceZ=off  EnableForce=on  TorqueResolutionFrame=World  EnableTorqueX=off  EnableTorqueY=off  EnableTorqueZ=off  EnableTorque=on
  Motion Sensor : Subsystem
  Rigid Transform (Setup CG) : sm_lib/Frames and Transforms/Rigid Transform  TranslationMethod=Cartesian  TranslationStandardOffset=0  TranslationLengthUnit=m  TranslationStandardAxis=+Z  TranslationCartesianOffset=body.cg  TranslationROffset=0  TranslationROffsetUnits=m  TranslationZOffset=0  TranslationZOffsetUnits=m  TranslationThetaOffset=0  TranslationThetaOffsetUnits=deg  RotationMethod=None  RotationAngleUnits=rad  RotationStandardAxis=+Y  RotationAngle=0.05  RotationArbitraryAxis=[0.57735026918962584 0.57735026918962584 0.57735026918962584]  FollAlignAxisA=+X  BaseAlignAxisA=+Y  FollAlignAxisB=+Y  BaseAlignAxisB=+Z  RotationSequenceAxes=FollowerAxes  RotationSequence=XYX  RotationSequenceAngles=[0 0 0]  RotationSequenceAnglesUnits=deg  RotationMatrix=[1 0 0; 0 1 0; 0 0 1]
  Rigid Transform (Setup Initial Disp) : sm_lib/Frames and Transforms/Rigid Transform  TranslationMethod=Cartesian  TranslationStandardOffset=0  TranslationLengthUnit=m  TranslationStandardAxis=+Z  TranslationCartesianOffset=body.initDisp.initLinDisp  TranslationROffset=0  TranslationROffsetUnits=m  TranslationZOffset=0  TranslationZOffsetUnits=m  TranslationThetaOffset=0  TranslationThetaOffsetUnits=deg  RotationMethod=ArbitraryAxis  RotationAngleUnits=rad  RotationStandardAxis=+Y  RotationAngle=body.initDisp.initAngularDispAngle  RotationArbitraryAxis=body.initDisp.initAngularDispAxis  FollAlignAxisA=+X  BaseAlignAxisA=+Y  FollAlignAxisB=+Y  BaseAlignAxisB=+Z  RotationSequenceAxes=FollowerAxes  RotationSequence=XYX  RotationSequenceAngles=[0 0 0]  RotationSequenceAnglesUnits=deg  RotationMatrix=[1 0 0; 0 1 0; 0 0 1]
  Selector : Selector  InputPortWidth=6  IndexOptions=Index vector (dialog)  Indices=[1:3]  OutputSizes=1
  Selector1 : Selector  InputPortWidth=6  IndexOptions=Index vector (dialog)  Indices=[4:6]  OutputSizes=1
  Simulink-PS Converter1 : nesl_utility/Simulink-PS Converter  PhysicalDomain=network_engine_domain  SubClassName=ps_input  LeftPortType=input  RightPortType=output  PseudoPeriodic=off  Frequencies=[]  NoiseDistribution=none  NoiseParameters=[]  Unit=1  AffineConversion=off  InputFiltering=off  SimscapeFilterOrder=1  InputFilterTimeConstant=0.001  UdotUserProvided=1
  Simulink-PS Converter2 : nesl_utility/Simulink-PS Converter  PhysicalDomain=network_engine_domain  SubClassName=ps_input  LeftPortType=input  RightPortType=output  PseudoPeriodic=off  Frequencies=[]  NoiseDistribution=none  NoiseParameters=[]  Unit=1  AffineConversion=off  InputFiltering=off  SimscapeFilterOrder=1  InputFilterTimeConstant=0.001  UdotUserProvided=1
  World Frame : sm_lib/Frames and Transforms/World Frame
  Conn Free Surface : PMIOPort  Port=1  Side=Right
  Response : Outport
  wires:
  Total Force/1 -> Selector1/1, Selector/1
  Selector/1 -> Simulink-PS Converter1/1
  Selector1/1 -> Simulink-PS Converter2/1
  Motion Sensor/1(Response) -> Response/1
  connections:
  External Force and Torque/LConn1 -- Simulink-PS Converter1/RConn1
  External Force and Torque/LConn2 -- Simulink-PS Converter2/RConn1
  Rigid Transform (Setup Initial Disp)/RConn1 -- Body Properties/RConn1 -- External Force and Torque/RConn1 -- Motion Sensor/RConn1
  Conn Free Surface/RConn1 -- Rigid Transform (Setup CG)/LConn1
  Rigid Transform (Setup Initial Disp)/LConn1 -- Rigid Transform (Setup CG)/RConn1
  World Frame/RConn1 -- Motion Sensor/LConn1

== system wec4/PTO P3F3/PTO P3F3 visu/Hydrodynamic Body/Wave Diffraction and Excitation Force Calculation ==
  Time : Inport
  Displacement : Inport  Port=2
  WaveElv : Inport  Port=3
  Add : Sum
  If2 : If  NumInputs=2  IfExpression=u1 < u2
  Linear Wave Excitation Force Variant Subsystem : Subsystem  Variant=on
  Merge1 : Merge
  No Ramp Function : Subsystem  TreatAsAtomicUnit=on
  Nonlinear FK Force Variant Subsystem : Subsystem  Variant=on
  Product : Product
  Ramp Function : Subsystem  TreatAsAtomicUnit=on
  Ramp Function Time : Constant  Value=simu.rampTime
  F_Excitation : Outport  PortDimensions=6
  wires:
  Nonlinear FK Force Variant Subsystem/1(Out1) -> Add/2
  Linear Wave Excitation Force Variant Subsystem/1(Out1) -> Add/1
  WaveElv/1 -> Nonlinear FK Force Variant Subsystem/3(In3)
  Displacement/1 -> Nonlinear FK Force Variant Subsystem/2(In2)
  Product/1 -> F_Excitation/1  "F_Excitation"
  Add/1 -> Product/2  "F_wave"
  Time/1 -> If2/1, Ramp Function/1(Time), Nonlinear FK Force Variant Subsystem/1(In1), Linear Wave Excitation Force Variant Subsystem/1(In1)
  Merge1/1 -> Product/1  "R"
  Ramp Function Time/1 -> If2/2
  If2/2 -> No Ramp Function/Action
  If2/1 -> Ramp Function/Action
  Ramp Function/1(R) -> Merge1/1
  No Ramp Function/1(R) -> Merge1/2

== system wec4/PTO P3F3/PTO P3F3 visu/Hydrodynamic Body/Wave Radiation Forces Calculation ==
  Velocity : Inport
  Acceleration : Inport  Port=2
  Time : Inport  Port=3
  Added Mass Matrix : Constant  Value=body.hydroForce.fAddedMass
  Product1 : Product  Multiplication=Matrix(*)
  SS CI and Constant-Damping-CoeVariant Subsystem : Subsystem  Variant=on
  Transport Delay : TransportDelay  DelayTime=10e-8
  F_RadiationDamping : Outport
  F_AddedMass : Outport  Port=2
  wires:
  Time/1 -> SS CI and Constant-Damping-CoeVariant Subsystem/2(In2)
  Acceleration/1 -> Transport Delay/1
  Transport Delay/1 -> Product1/2
  SS CI and Constant-Damping-CoeVariant Subsystem/1(Out1) -> F_RadiationDamping/1  "F_RadiationDamping"
  Velocity/1 -> SS CI and Constant-Damping-CoeVariant Subsystem/1(In1)
  Product1/1 -> F_AddedMass/1  "F_AddedMass"
  Added Mass Matrix/1 -> Product1/1

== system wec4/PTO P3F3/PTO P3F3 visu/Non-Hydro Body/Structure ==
  Total Force : Inport
  Body Properties : sm_lib/Body Elements/Solid  InertiaType=Custom  Mass=body.mass  MassUnits=kg  CenterOfMass=[0 0 0]  CenterOfMassUnits=m  MomentsOfInertia=body.momOfInertia  MomentsOfInertiaUnits=kg*m^2  ProductsOfInertia=[0 0 0]  ProductsOfInertiaUnits=kg*m^2  DensityBased=on  Density=1000  DensityUnits=kg/(m^3)  DoExposeReferenceFrame=on  SerializedFrames=<Frames/>  GraphicType=FromGeometry  MarkerShape=Sphere  MarkerSize=10  MarkerSizeUnits=m  GraphicVisPropType=SimpleVisualProperties  GraphicDiffuseColor=body.viz.color  GraphicSpecularColor=[0.5 0.5 0.5 1.0]  GraphicAmbientColor=[0.15 0.15 0.15 1.0]  GraphicEmissiveColor=[0.0 0.0 0.0 1.0]  GraphicShininess=75  GraphicOpacity=body.viz.opacity  GeometryShape=FromFile  RectangleSize=[1 1]  RectangleSizeUnits=m  BrickDimensions=[1 1 1]  BrickDimensionUnits=m  CylinderRadius=1  CylinderRadiusUnits=m  CylinderLength=1  CylinderLengthUnits=m  SphereRadius=1  SphereRadiusUnits=m  EllipsoidRadii=[1 1 1]  EllipsoidRadiiUnits=m  ExtrusionCrossSection=[1 1; -1 1; -1 -1; 1 -1]  ExtrusionCrossSectionUnits=m  ExtrusionLength=1  ExtrusionLengthUnits=m  PolygonNumSides=3  PolygonOuterRadius=1  PolygonOuterRadiusUnits=m  ExtGeomFileType=STL  ExtGeomFileName=.\geometry\pto_visu.stl  ExtGeomFileUnits=m  RevolutionCrossSection=[1 1; 1 -1; 2 -1; 2 1]  RevolutionCrossSectionUnits=m  RevolutionExtent=Full  RevolutionAngle=180  RevolutionAngleUnits=deg
  External Force and Torque : sm_lib/Forces and Torques/External Force and Torque  ForceResolutionFrame=World  EnableForceX=off  EnableForceY=off  EnableForceZ=off  EnableForce=on  TorqueResolutionFrame=World  EnableTorqueX=off  EnableTorqueY=off  EnableTorqueZ=off  EnableTorque=on
  Motion Sensor : Subsystem
  Rigid Transform (Setup CG) : sm_lib/Frames and Transforms/Rigid Transform  TranslationMethod=Cartesian  TranslationStandardOffset=0  TranslationLengthUnit=m  TranslationStandardAxis=+Z  TranslationCartesianOffset=body.cg  TranslationROffset=0  TranslationROffsetUnits=m  TranslationZOffset=0  TranslationZOffsetUnits=m  TranslationThetaOffset=0  TranslationThetaOffsetUnits=deg  RotationMethod=None  RotationAngleUnits=rad  RotationStandardAxis=+Y  RotationAngle=0.05  RotationArbitraryAxis=[0.57735026918962584 0.57735026918962584 0.57735026918962584]  FollAlignAxisA=+X  BaseAlignAxisA=+Y  FollAlignAxisB=+Y  BaseAlignAxisB=+Z  RotationSequenceAxes=FollowerAxes  RotationSequence=XYX  RotationSequenceAngles=[0 0 0]  RotationSequenceAnglesUnits=deg  RotationMatrix=[1 0 0; 0 1 0; 0 0 1]
  Rigid Transform (Setup Initial Disp) : sm_lib/Frames and Transforms/Rigid Transform  TranslationMethod=Cartesian  TranslationStandardOffset=0  TranslationLengthUnit=m  TranslationStandardAxis=+Z  TranslationCartesianOffset=body.initDisp.initLinDisp  TranslationROffset=0  TranslationROffsetUnits=m  TranslationZOffset=0  TranslationZOffsetUnits=m  TranslationThetaOffset=0  TranslationThetaOffsetUnits=deg  RotationMethod=ArbitraryAxis  RotationAngleUnits=rad  RotationStandardAxis=+Y  RotationAngle=body.initDisp.initAngularDispAngle  RotationArbitraryAxis=body.initDisp.initAngularDispAxis  FollAlignAxisA=+X  BaseAlignAxisA=+Y  FollAlignAxisB=+Y  BaseAlignAxisB=+Z  RotationSequenceAxes=FollowerAxes  RotationSequence=XYX  RotationSequenceAngles=[0 0 0]  RotationSequenceAnglesUnits=deg  RotationMatrix=[1 0 0; 0 1 0; 0 0 1]
  Selector : Selector  InputPortWidth=6  IndexOptions=Index vector (dialog)  Indices=[1:3]  OutputSizes=1
  Selector1 : Selector  InputPortWidth=6  IndexOptions=Index vector (dialog)  Indices=[4:6]  OutputSizes=1
  Simulink-PS Converter1 : nesl_utility/Simulink-PS Converter  PhysicalDomain=network_engine_domain  SubClassName=ps_input  LeftPortType=input  RightPortType=output  PseudoPeriodic=off  Frequencies=[]  NoiseDistribution=none  NoiseParameters=[]  Unit=1  AffineConversion=off  InputFiltering=off  SimscapeFilterOrder=1  InputFilterTimeConstant=0.001  UdotUserProvided=1
  Simulink-PS Converter2 : nesl_utility/Simulink-PS Converter  PhysicalDomain=network_engine_domain  SubClassName=ps_input  LeftPortType=input  RightPortType=output  PseudoPeriodic=off  Frequencies=[]  NoiseDistribution=none  NoiseParameters=[]  Unit=1  AffineConversion=off  InputFiltering=off  SimscapeFilterOrder=1  InputFilterTimeConstant=0.001  UdotUserProvided=1
  World Frame : sm_lib/Frames and Transforms/World Frame
  Conn Free Surface : PMIOPort  Port=1  Side=Right
  Response : Outport
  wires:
  Total Force/1 -> Selector1/1, Selector/1
  Selector/1 -> Simulink-PS Converter1/1
  Selector1/1 -> Simulink-PS Converter2/1
  Motion Sensor/1(Response) -> Response/1
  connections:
  External Force and Torque/LConn1 -- Simulink-PS Converter1/RConn1
  External Force and Torque/LConn2 -- Simulink-PS Converter2/RConn1
  Rigid Transform (Setup Initial Disp)/RConn1 -- Body Properties/RConn1 -- External Force and Torque/RConn1 -- Motion Sensor/RConn1
  Conn Free Surface/RConn1 -- Rigid Transform (Setup CG)/LConn1
  Rigid Transform (Setup Initial Disp)/LConn1 -- Rigid Transform (Setup CG)/RConn1
  World Frame/RConn1 -- Motion Sensor/LConn1

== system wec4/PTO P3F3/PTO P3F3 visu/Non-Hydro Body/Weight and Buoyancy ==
  Add1 : Sum  Inputs=+-
  Assignment (Add Net Bouyancy Force to Z-Direction) : Assignment  IndexOptions=Index vector (dialog)  Indices=3  OutputSizes=1
  Body Mass : Constant  Value=body.mass
  Constant1 : Constant  Value=[0 0 0 0 0 0]
  Gravity : Constant  Value=simu.g
  Product : Product
  Product1 : Product  Inputs=3
  Volume : Constant  Value=body.dispVol
  Water Density : Constant  Value=simu.rho
  Out1 : Outport
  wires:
  Add1/1 -> Assignment (Add Net Bouyancy Force to Z-Direction)/2
  Product1/1 -> Add1/2  "F_Buoyancy"
  Product/1 -> Add1/1  "F_Gravity"
  Water Density/1 -> Product1/1  "rho"
  Gravity/1 -> Product/1, Product1/2  "g"
  Volume/1 -> Product1/3  "Vol"
  Assignment (Add Net Bouyancy Force to Z-Direction)/1 -> Out1/1  "F_Restoring"
  Constant1/1 -> Assignment (Add Net Bouyancy Force to Z-Direction)/1
  Body Mass/1 -> Product/2  "m"

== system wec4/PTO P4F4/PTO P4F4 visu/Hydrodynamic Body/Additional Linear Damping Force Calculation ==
  Velocity : Inport
  Additional Linear Damping Matrix (diagonal) : Constant  Value=body.hydroForce.linearDamping
  Product1 : Product  Multiplication=Matrix(*)
  F_LinearDamping : Outport
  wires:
  Velocity/1 -> Product1/2  "v"
  Product1/1 -> F_LinearDamping/1  "F_LinearDamping"
  Additional Linear Damping Matrix (diagonal)/1 -> Product1/1  "C"

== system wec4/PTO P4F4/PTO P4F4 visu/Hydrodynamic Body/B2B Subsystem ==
  note: 1) Add Subsystem or Model blocks as valid variant choices. 2) You cannot connect blocks at this level. At simulation, connectivity is automatically determined, based on the active variant and port name matching.
  vel_in : Inport
  acc_in : Inport  Port=2
  B2B : Subsystem  VariantControl=sv_B2B
  noB2B : Subsystem  VariantControl=sv_noB2B
  vel : Outport
  acc : Outport  Port=2

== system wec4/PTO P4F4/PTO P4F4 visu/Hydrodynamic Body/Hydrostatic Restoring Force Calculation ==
  Displacement : Inport
  Wave Elv : Inport  Port=2
  Add : Sum  Inputs=+-
  Center of Gravity : Constant  Value=body.cg
  Constant : Constant  Value=[0 0 0]
  Linear and Nonlinear Restoring Force Variant Subsystem : Subsystem  Variant=on
  Mux : Mux  Inputs=2
  F_Restoring : Outport
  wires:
  Add/1 -> Linear and Nonlinear Restoring Force Variant Subsystem/1(In1)  "x_cg"
  Wave Elv/1 -> Linear and Nonlinear Restoring Force Variant Subsystem/2(In2)
  Constant/1 -> Mux/2
  Center of Gravity/1 -> Mux/1  "cg"
  Mux/1 -> Add/2
  Linear and Nonlinear Restoring Force Variant Subsystem/1(Out1) -> F_Restoring/1  "F_Restoring"
  Displacement/1 -> Add/1  "x"
